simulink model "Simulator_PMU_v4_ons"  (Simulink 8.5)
settings: Solver=FixedStepDiscrete  StartTime=0.0  StopTime=5  FixedStep=1/(60*32)  RelTol=1e-3
undefined symbols (not defined in the file or in its folder): complex, j
libraries: dspxfrm3 x3

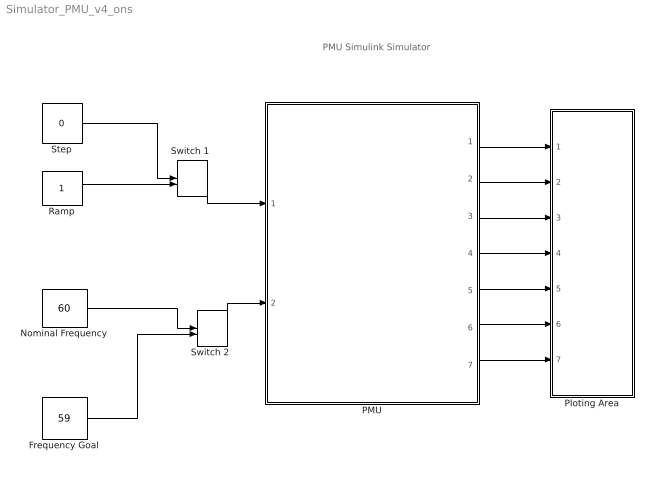
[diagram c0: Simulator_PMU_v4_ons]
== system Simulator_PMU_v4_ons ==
  note: PMU Simulink Simulator
  Frequency Goal : Constant  Value=59
  Nominal Frequency : Constant  Value=60
  PMU : Subsystem
  Ploting Area : Subsystem
  Ramp : Constant
  Step : Constant  Value=0
  "Switch 1 " : ManualSwitch
  "Switch 2 " : ManualSwitch  CurrentSetting=0
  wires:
  PMU/1(SP_MF) -> Ploting Area/1(SP_MF)
  PMU/2(SP_MnF) -> Ploting Area/2(SP_MnF)
  PMU/4(PS_Md) -> Ploting Area/4(PS_Md)
  PMU/6(PS_Ad) -> Ploting Area/6(PS_Ad)
  Step/1 -> "Switch 1 "/1
  Ramp/1 -> "Switch 1 "/2
  "Switch 2 "/1 -> PMU/2(Frequency Goal)
  PMU/3(PS_M) -> Ploting Area/3(PS_M)
  PMU/5(PS_A) -> Ploting Area/5(PS_A)
  PMU/7(Frequency  Deviation) -> Ploting Area/7(FD)
  Nominal Frequency/1 -> "Switch 2 "/1
  Frequency Goal/1 -> "Switch 2 "/2
  "Switch 1 "/1 -> PMU/1(Disturbance)

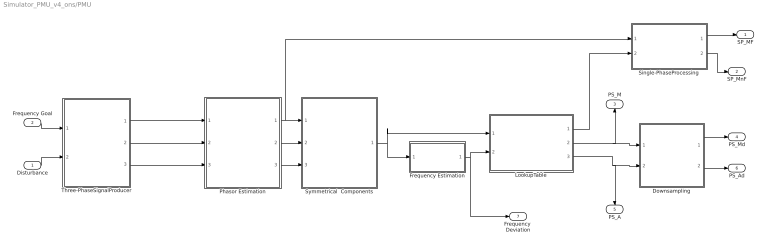
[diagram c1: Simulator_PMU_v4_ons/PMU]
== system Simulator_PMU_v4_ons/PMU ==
  Disturbance : Inport
  Frequency Goal : Inport  Port=2
  Downsampling : Subsystem
  Frequency Estimation : Subsystem
  LookupTable : Subsystem
  Phasor Estimation : Subsystem
  Single-PhaseProcessing : Subsystem
  Symmetrical  Components : Subsystem
  Three-PhaseSignalProducer : Subsystem
  SP_MF : Outport
  SP_MnF : Outport  Port=2
  PS_M : Outport  Port=3
  PS_Md : Outport  Port=4
  PS_A : Outport  Port=5
  PS_Ad : Outport  Port=6
  Frequency  Deviation : Outport  Port=7
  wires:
  Phasor Estimation/1(Phasor A) -> Single-PhaseProcessing/1(Phasor A), Symmetrical  Components/1(Phasor A)
  Symmetrical  Components/1(P_PS) -> Frequency Estimation/1(P_PS), LookupTable/1(P_ PS)
  LookupTable/2(PS_M) -> Downsampling/1(PS_M), PS_M/1
  LookupTable/3(PS_A) -> Downsampling/2(PS_A), PS_A/1
  Frequency Estimation/1(FD) -> LookupTable/2(FD), Frequency  Deviation/1
  LookupTable/1(CF) -> Single-PhaseProcessing/2(CF)
  Phasor Estimation/2(Phasor B) -> Symmetrical  Components/2(Phasor B)
  Phasor Estimation/3(Phasor C) -> Symmetrical  Components/3(Phasor C)
  Single-PhaseProcessing/1(SP_MF) -> SP_MF/1
  Single-PhaseProcessing/2(SP_MnF) -> SP_MnF/1
  Downsampling/1(" PS_Md") -> PS_Md/1
  Frequency Goal/1 -> Three-PhaseSignalProducer/1(Frequency)
  Downsampling/2(PS_Ad) -> PS_Ad/1
  Disturbance/1 -> Three-PhaseSignalProducer/2(Type)
  Three-PhaseSignalProducer/1(Phase A) -> Phasor Estimation/1(" Phase A")
  Three-PhaseSignalProducer/2(Phase B) -> Phasor Estimation/2(Phase B)
  Three-PhaseSignalProducer/3(Phase C) -> Phasor Estimation/3(Phase C)

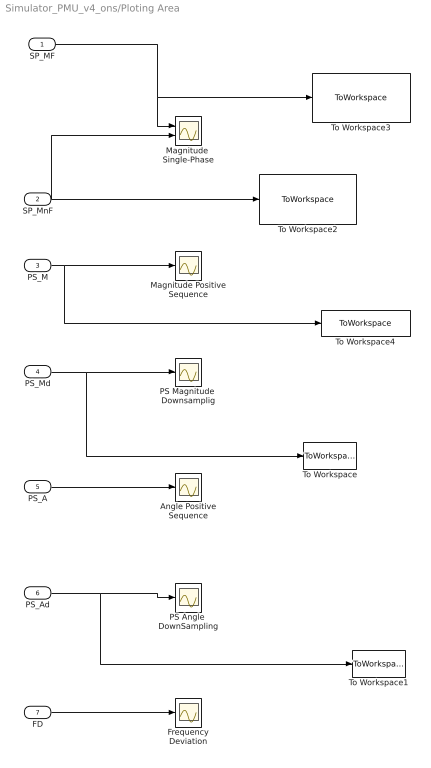
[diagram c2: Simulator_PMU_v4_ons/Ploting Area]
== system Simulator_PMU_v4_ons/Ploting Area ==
  SP_MF : Inport
  SP_MnF : Inport  Port=2
  PS_M : Inport  Port=3
  PS_Md : Inport  Port=4
  PS_A : Inport  Port=5
  PS_Ad : Inport  Port=6
  FD : Inport  Port=7
  Angle Positive Sequence : Scope
  Frequency Deviation : Scope
  Magnitude  Single-Phase : Scope  NumInputPorts=2
  Magnitude Positive Sequence : Scope
  PS Angle  DownSampling : Scope
  PS Magnitude  Downsamplig : Scope
  To Workspace : ToWorkspace  VariableName=simoutmagd  SaveFormat=Structure With Time  SampleTime=-1
  To Workspace1 : ToWorkspace  VariableName=simoutangd  SaveFormat=Structure With Time  SampleTime=-1
  To Workspace2 : ToWorkspace  VariableName=sp_mag_f  SaveFormat=Structure  SampleTime=-1
  To Workspace3 : ToWorkspace  VariableName=sp_mag  SaveFormat=Structure  SampleTime=-1
  To Workspace4 : ToWorkspace  VariableName=ps_magnitude  SaveFormat=Structure With Time  SampleTime=-1
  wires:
  SP_MF/1 -> Magnitude  Single-Phase/1, To Workspace3/1
  SP_MnF/1 -> Magnitude  Single-Phase/2, To Workspace2/1
  PS_M/1 -> Magnitude Positive Sequence/1, To Workspace4/1
  PS_Md/1 -> PS Magnitude  Downsamplig/1, To Workspace/1
  PS_A/1 -> Angle Positive Sequence/1
  PS_Ad/1 -> PS Angle  DownSampling/1, To Workspace1/1
  FD/1 -> Frequency Deviation/1

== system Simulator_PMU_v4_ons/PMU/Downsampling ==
  PS_M : Inport
  PS_A : Inport  Port=2
  Downsample A : DownSample  N=32  RateOptions=Allow multirate processing
  Downsample M : DownSample  N=32  RateOptions=Allow multirate processing
  Gain : Gain  Gain=180/pi
  " PS_Md" : Outport
  PS_Ad : Outport  Port=2
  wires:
  Downsample M/1 -> " PS_Md"/1
  PS_M/1 -> Downsample M/1
  PS_A/1 -> Downsample A/1
  Gain/1 -> PS_Ad/1
  Downsample A/1 -> Gain/1

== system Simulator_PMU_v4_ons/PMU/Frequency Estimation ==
  P_PS : Inport
  Complex to Magnitude-Angle : ComplexToMagnitudeAngle  Output=Angle
  Frequency Buffer : Buffer  N=32*2+1  V=32*2-1  TreatMby1Signals=One channel
  Frequency Datalog : ToWorkspace  VariableName=simoutf  SampleTime=-1
  Frequency  Estimation : MATLABFcn  MATLABFcn=freq_angle  Output1D=off
  FD : Outport
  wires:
  Frequency Buffer/1 -> Frequency  Estimation/1
  Frequency  Estimation/1 -> Frequency Datalog/1, FD/1
  Complex to Magnitude-Angle/1 -> Frequency Buffer/1
  P_PS/1 -> Complex to Magnitude-Angle/1

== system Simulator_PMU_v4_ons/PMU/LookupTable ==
  P_ PS : Inport
  FD : Inport  Port=2
  Complex to Magnitude-Angle : ComplexToMagnitudeAngle
  Divide : Product  Inputs=*/
  P_n Estimation : Subsystem
  Reshape : Reshape
  CF : Outport
  PS_M : Outport  Port=2
  PS_A : Outport  Port=3
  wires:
  Divide/1 -> Complex to Magnitude-Angle/1
  FD/1 -> Reshape/1
  Complex to Magnitude-Angle/1 -> PS_M/1
  Complex to Magnitude-Angle/2 -> PS_A/1
  P_ PS/1 -> Divide/1
  P_n Estimation/1(P_n) -> Divide/2, CF/1
  Reshape/1 -> P_n Estimation/1(Frequency Deviation)

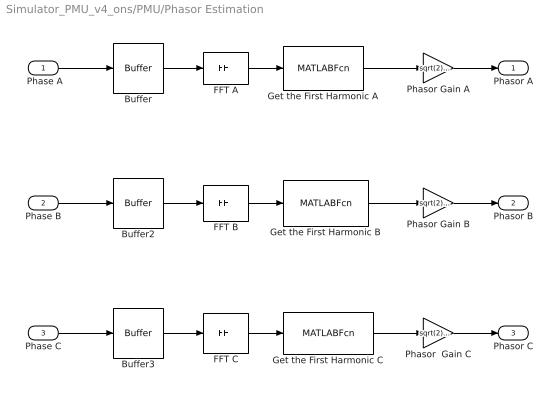
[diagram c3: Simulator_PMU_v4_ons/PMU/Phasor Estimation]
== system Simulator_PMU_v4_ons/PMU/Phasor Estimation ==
  " Phase A" : Inport
  Phase B : Inport  Port=2
  Phase C : Inport  Port=3
  Buffer : Buffer  N=32  V=31  TreatMby1Signals=One channel
  Buffer2 : Buffer  N=32  V=31  TreatMby1Signals=One channel
  Buffer3 : Buffer  N=32  V=31  TreatMby1Signals=One channel
  FFT A : dspxfrm3/FFT  CompMethod=Table lookup  TableOpt=HYBRID  TableOptActive=Speed  BitRevOrder=off  InheritFFTLength=on  FFTLength=31  WrapInput=on  RowConvenienceOn=on  FFTImplementation=Auto  SkipNorm=off  firstCoeffDataTypeStr=Inherit: Same word length as input  firstCoeffLastDataTypeStr=Inherit: Same word length as input  outputMin=[]  outputMax=[]  roundingMode=Round  overflowMode=off
  FFT B : dspxfrm3/FFT  CompMethod=Table lookup  TableOpt=HYBRID  TableOptActive=Speed  BitRevOrder=off  InheritFFTLength=on  FFTLength=32  WrapInput=on  RowConvenienceOn=on  FFTImplementation=Auto  SkipNorm=off  firstCoeffDataTypeStr=Inherit: Same word length as input  firstCoeffLastDataTypeStr=Inherit: Same word length as input  outputMin=[]  outputMax=[]  roundingMode=Round  overflowMode=off
  FFT C : dspxfrm3/FFT  CompMethod=Table lookup  TableOpt=HYBRID  TableOptActive=Speed  BitRevOrder=off  InheritFFTLength=on  FFTLength=32  WrapInput=on  RowConvenienceOn=on  FFTImplementation=Auto  SkipNorm=off  firstCoeffDataTypeStr=Inherit: Same word length as input  firstCoeffLastDataTypeStr=Inherit: Same word length as input  outputMin=[]  outputMax=[]  roundingMode=Round  overflowMode=off
  Get the First Harmonic A : MATLABFcn  MATLABFcn=u(2,1,1)  OutputSignalType=complex
  Get the First Harmonic B : MATLABFcn  MATLABFcn=u(2,1,1)  OutputSignalType=complex
  Get the First Harmonic C : MATLABFcn  MATLABFcn=u(2,1,1)  OutputSignalType=complex
  Phasor Gain A : Gain  Gain=sqrt(2)/32
  Phasor Gain B : Gain  Gain=sqrt(2)/32
  Phasor  Gain C : Gain  Gain=sqrt(2)/32
  Phasor A : Outport
  Phasor B : Outport  Port=2
  Phasor C : Outport  Port=3
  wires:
  FFT A/1 -> Get the First Harmonic A/1
  Buffer/1 -> FFT A/1
  Get the First Harmonic A/1 -> Phasor Gain A/1
  FFT B/1 -> Get the First Harmonic B/1
  Buffer2/1 -> FFT B/1
  Get the First Harmonic B/1 -> Phasor Gain B/1
  FFT C/1 -> Get the First Harmonic C/1
  Buffer3/1 -> FFT C/1
  Get the First Harmonic C/1 -> Phasor  Gain C/1
  " Phase A"/1 -> Buffer/1
  Phasor Gain A/1 -> Phasor A/1
  Phase B/1 -> Buffer2/1
  Phasor Gain B/1 -> Phasor B/1
  Phase C/1 -> Buffer3/1
  Phasor  Gain C/1 -> Phasor C/1

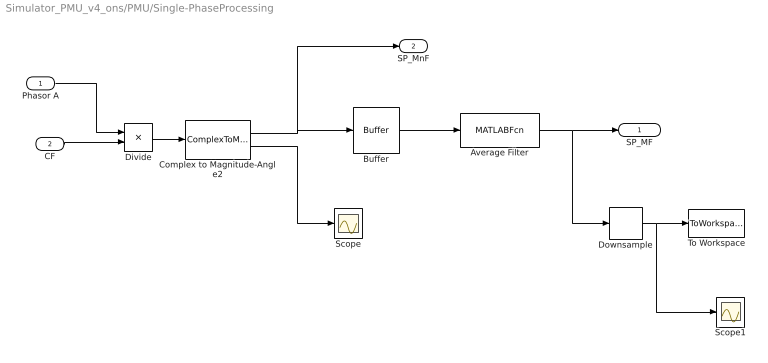
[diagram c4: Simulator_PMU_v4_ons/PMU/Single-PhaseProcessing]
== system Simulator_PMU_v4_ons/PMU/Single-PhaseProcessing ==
  Phasor A : Inport
  CF : Inport  Port=2
  Average Filter : MATLABFcn  MATLABFcn=( u(1)+u(6)+u(12) )/3  Output1D=off
  Buffer : Buffer  N=32  V=31  TreatMby1Signals=One channel
  Complex to Magnitude-Angle2 : ComplexToMagnitudeAngle
  Divide : Product  Inputs=*/
  Downsample : DownSample  N=32  RateOptions=Allow multirate processing
  Scope : Scope
  Scope1 : Scope
  To Workspace : ToWorkspace  VariableName=single  SaveFormat=Structure  SampleTime=-1
  SP_MF : Outport
  SP_MnF : Outport  Port=2
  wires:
  Phasor A/1 -> Divide/1
  CF/1 -> Divide/2
  Complex to Magnitude-Angle2/2 -> Scope/1
  Complex to Magnitude-Angle2/1 -> Buffer/1, SP_MnF/1
  Buffer/1 -> Average Filter/1
  Divide/1 -> Complex to Magnitude-Angle2/1
  Average Filter/1 -> SP_MF/1, Downsample/1
  Downsample/1 -> To Workspace/1, Scope1/1

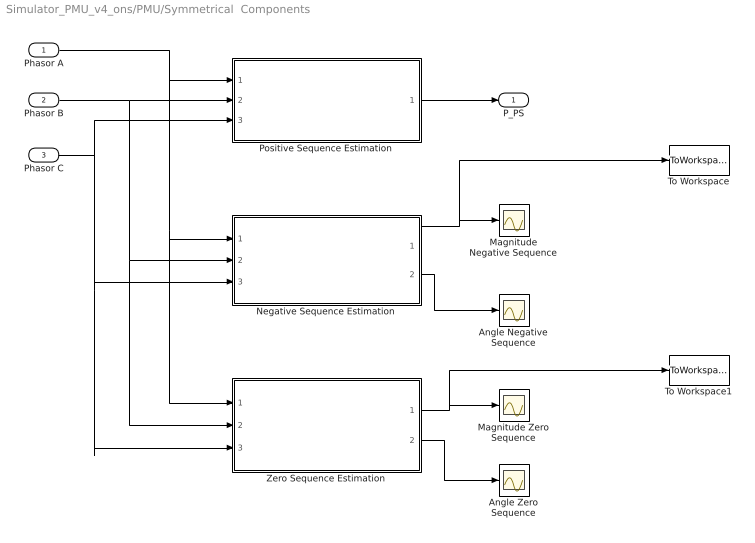
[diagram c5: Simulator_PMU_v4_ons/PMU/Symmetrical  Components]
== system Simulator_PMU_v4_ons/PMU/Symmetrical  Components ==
  Phasor A : Inport
  Phasor B : Inport  Port=2
  Phasor C : Inport  Port=3
  Angle Negative Sequence : Scope
  Angle Zero Sequence : Scope
  Magnitude Negative Sequence : Scope
  Magnitude Zero Sequence : Scope
  Negative Sequence Estimation : Subsystem
  Positive Sequence Estimation : Subsystem
  To Workspace : ToWorkspace  VariableName=negative  SaveFormat=Structure  SampleTime=-1
  To Workspace1 : ToWorkspace  VariableName=zero  SaveFormat=Structure  SampleTime=-1
  Zero Sequence Estimation : Subsystem
  P_PS : Outport
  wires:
  Phasor C/1 -> Zero Sequence Estimation/3(Phasor C), Negative Sequence Estimation/3(Phasor C), Positive Sequence Estimation/3(Phasor C)
  Phasor B/1 -> Zero Sequence Estimation/2(Phasor B), Negative Sequence Estimation/2(Phasor B), Positive Sequence Estimation/2(Phasor B)
  Negative Sequence Estimation/2(Angle) -> Angle Negative Sequence/1
  Negative Sequence Estimation/1(Magnitude) -> Magnitude Negative Sequence/1, To Workspace/1
  Zero Sequence Estimation/2(Angle) -> Angle Zero Sequence/1
  Zero Sequence Estimation/1(Magnitude) -> Magnitude Zero Sequence/1, To Workspace1/1
  Phasor A/1 -> Positive Sequence Estimation/1(Phasor A), Negative Sequence Estimation/1(Phasor A), Zero Sequence Estimation/1(Phasor A)
  Positive Sequence Estimation/1(Positive Sequence) -> P_PS/1

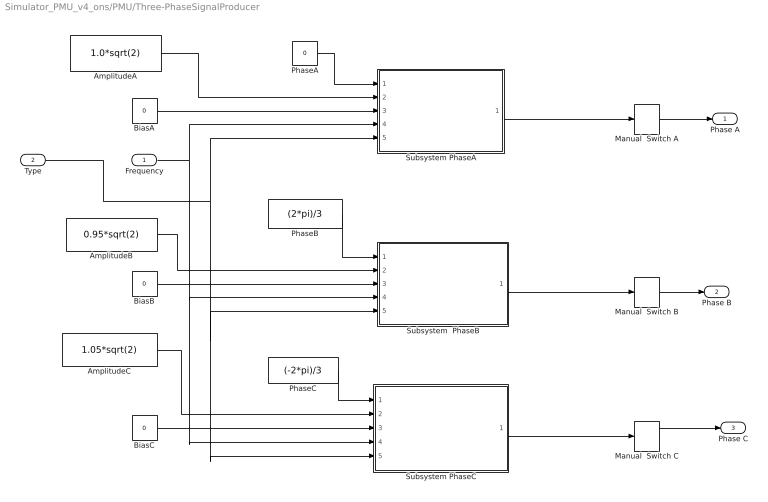
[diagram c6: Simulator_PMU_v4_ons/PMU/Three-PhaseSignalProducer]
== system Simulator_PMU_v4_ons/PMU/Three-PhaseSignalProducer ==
  Frequency : Inport
  Type : Inport  Port=2
  AmplitudeA : Constant  Value=1.0*sqrt(2)
  AmplitudeB : Constant  Value=0.95*sqrt(2)
  AmplitudeC : Constant  Value=1.05*sqrt(2)
  BiasA : Constant  Value=0
  BiasB : Constant  Value=0
  BiasC : Constant  Value=0
  Manual  Switch A : ManualSwitch
  Manual  Switch B : ManualSwitch
  Manual  Switch C : ManualSwitch
  PhaseA : Constant  Value=0
  PhaseB : Constant  Value=(2*pi)/3
  PhaseC : Constant  Value=(-2*pi)/3
  Subsystem PhaseA : Subsystem
  Subsystem PhaseC : Subsystem
  Subsystem  PhaseB : Subsystem
  Phase A : Outport
  Phase B : Outport  Port=2
  Phase C : Outport  Port=3
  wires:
  AmplitudeB/1 -> Subsystem  PhaseB/2(Amplitude)
  BiasB/1 -> Subsystem  PhaseB/3(Bias)
  PhaseB/1 -> Subsystem  PhaseB/1(Phase)
  AmplitudeC/1 -> Subsystem PhaseC/2(Amplitude)
  BiasC/1 -> Subsystem PhaseC/3(Bias)
  PhaseC/1 -> Subsystem PhaseC/1(Phase)
  BiasA/1 -> Subsystem PhaseA/3(Bias)
  PhaseA/1 -> Subsystem PhaseA/1(Phase)
  AmplitudeA/1 -> Subsystem PhaseA/2(Amplitude)
  Frequency/1 -> Subsystem PhaseA/4(Frequency), Subsystem  PhaseB/4(Frequency), Subsystem PhaseC/4(Frequency)
  Type/1 -> Subsystem PhaseA/5(Ramp/Step), Subsystem  PhaseB/5(Ramp/Step), Subsystem PhaseC/5(Ramp/Step)
  Subsystem PhaseC/1(Signal) -> Manual  Switch C/1
  Manual  Switch C/1 -> Phase C/1
  Manual  Switch B/1 -> Phase B/1
  Subsystem  PhaseB/1(Signal) -> Manual  Switch B/1
  Manual  Switch A/1 -> Phase A/1
  Subsystem PhaseA/1("Signal ") -> Manual  Switch A/1

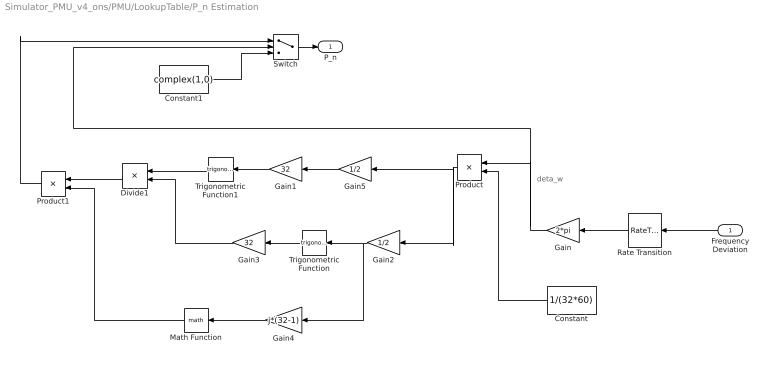
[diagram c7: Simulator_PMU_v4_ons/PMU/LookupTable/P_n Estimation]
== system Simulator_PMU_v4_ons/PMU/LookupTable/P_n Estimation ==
  note: deta_w
  Frequency Deviation : Inport
  Constant : Constant  Value=1/(32*60)
  Constant1 : Constant  Value=complex(1,0)  VectorParams1D=off
  Divide1 : Product  Inputs=*/
  Gain : Gain  Gain=2*pi  SampleTime=1/(32*60)
  Gain1 : Gain  Gain=32
  Gain2 : Gain  Gain=1/2
  Gain3 : Gain  Gain=32
  Gain4 : Gain  Gain=j*(32-1)
  Gain5 : Gain  Gain=1/2
  Math Function : Math
  Product : Product
  Product1 : Product
  Rate Transition : RateTransition  OutPortSampleTime=1/(32*60)
  Switch : Switch  Criteria=u2 ~= 0
  Trigonometric Function : Trigonometry
  Trigonometric Function1 : Trigonometry
  P_n : Outport
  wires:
  Gain/1 -> Product/1, Switch/2
  Constant/1 -> Product/2
  Product/1 -> Gain2/1, Gain5/1
  Gain2/1 -> Trigonometric Function/1, Gain4/1
  Trigonometric Function/1 -> Gain3/1
  Gain1/1 -> Trigonometric Function1/1
  Gain3/1 -> Divide1/2
  Trigonometric Function1/1 -> Divide1/1
  Gain4/1 -> Math Function/1
  Product1/1 -> Switch/1
  Constant1/1 -> Switch/3
  Gain5/1 -> Gain1/1
  Rate Transition/1 -> Gain/1
  Divide1/1 -> Product1/1
  Math Function/1 -> Product1/2
  Switch/1 -> P_n/1
  Frequency Deviation/1 -> Rate Transition/1

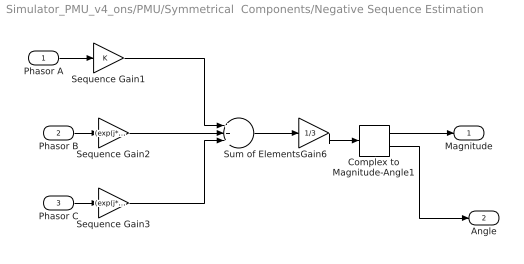
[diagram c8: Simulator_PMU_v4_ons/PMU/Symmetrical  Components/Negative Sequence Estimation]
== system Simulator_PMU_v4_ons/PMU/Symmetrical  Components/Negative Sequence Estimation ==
  Phasor A : Inport
  Phasor B : Inport  Port=2
  Phasor C : Inport  Port=3
  Complex to Magnitude-Angle1 : ComplexToMagnitudeAngle
  Gain6 : Gain  Gain=1/3  SampleTime=1/(32*60)
  Sequence Gain1 : Gain
  Sequence Gain2 : Gain  Gain=(exp(j*2*pi/3))
  Sequence Gain3 : Gain  Gain=(exp(j*2*pi/3))^2
  Sum of Elements : Sum  Inputs=+++
  Magnitude : Outport
  Angle : Outport  Port=2
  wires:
  Sequence Gain1/1 -> Sum of Elements/1
  Sequence Gain2/1 -> Sum of Elements/2
  Sequence Gain3/1 -> Sum of Elements/3
  Sum of Elements/1 -> Gain6/1
  Phasor A/1 -> Sequence Gain1/1
  Gain6/1 -> Complex to Magnitude-Angle1/1
  Phasor B/1 -> Sequence Gain2/1
  Phasor C/1 -> Sequence Gain3/1
  Complex to Magnitude-Angle1/1 -> Magnitude/1
  Complex to Magnitude-Angle1/2 -> Angle/1

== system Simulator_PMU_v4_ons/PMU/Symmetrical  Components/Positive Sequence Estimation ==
  Phasor A : Inport
  Phasor B : Inport  Port=2
  Phasor C : Inport  Port=3
  Gain6 : Gain  Gain=1/3  SampleTime=1/(32*60)
  Sequence Gain1 : Gain
  Sequence Gain2 : Gain  Gain=(exp(j*2*pi/3))^2
  Sequence Gain3 : Gain  Gain=exp(j*2*pi/3)
  Sum of Elements : Sum  Inputs=+++
  Positive Sequence : Outport
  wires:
  Sequence Gain1/1 -> Sum of Elements/1
  Sequence Gain2/1 -> Sum of Elements/2
  Sequence Gain3/1 -> Sum of Elements/3
  Sum of Elements/1 -> Gain6/1
  Phasor A/1 -> Sequence Gain1/1
  Gain6/1 -> Positive Sequence/1
  Phasor B/1 -> Sequence Gain2/1
  Phasor C/1 -> Sequence Gain3/1

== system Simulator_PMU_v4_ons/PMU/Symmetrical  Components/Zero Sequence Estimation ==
  Phasor A : Inport
  Phasor B : Inport  Port=2
  Phasor C : Inport  Port=3
  Complex to Magnitude-Angle1 : ComplexToMagnitudeAngle
  Gain6 : Gain  Gain=1/3  SampleTime=1/(32*60)
  Sequence Gain1 : Gain
  Sequence Gain2 : Gain
  Sequence Gain3 : Gain
  Sum of Elements : Sum  Inputs=+++
  Magnitude : Outport
  Angle : Outport  Port=2
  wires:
  Sequence Gain1/1 -> Sum of Elements/1
  Sequence Gain2/1 -> Sum of Elements/2
  Sequence Gain3/1 -> Sum of Elements/3
  Sum of Elements/1 -> Gain6/1
  Phasor A/1 -> Sequence Gain1/1
  Gain6/1 -> Complex to Magnitude-Angle1/1
  Phasor B/1 -> Sequence Gain2/1
  Phasor C/1 -> Sequence Gain3/1
  Complex to Magnitude-Angle1/1 -> Magnitude/1
  Complex to Magnitude-Angle1/2 -> Angle/1

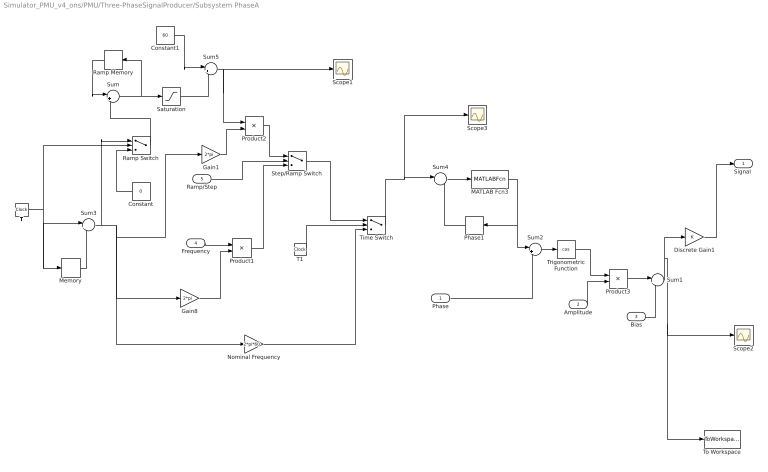
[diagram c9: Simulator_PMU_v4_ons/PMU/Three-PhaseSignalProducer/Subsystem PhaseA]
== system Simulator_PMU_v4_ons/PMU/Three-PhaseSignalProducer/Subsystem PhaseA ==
  Phase : Inport
  Amplitude : Inport  Port=2
  Bias : Inport  Port=3
  Frequency : Inport  Port=4
  Ramp/Step : Inport  Port=5
  Constant : Constant  Value=0
  Constant1 : Constant  Value=60
  Discrete Gain1 : Gain  SampleTime=1/(32*60)
  Gain1 : Gain  Gain=2*pi
  Gain8 : Gain  Gain=2*pi
  MATLAB Fcn3 : MATLABFcn  MATLABFcn=rem(u,2*pi)
  Memory : Memory
  Nominal Frequency : Gain  Gain=2*pi*60
  Phase1 : Memory  X0=-(2*pi)/32  LinearizeMemory=on
  Product1 : Product
  Product2 : Product
  Product3 : Product
  Ramp Memory : Memory
  Ramp Switch : Switch  Threshold=2
  Saturation : Saturate  UpperLimit=1  LowerLimit=-1
  Scope1 : Scope
  Scope2 : Scope
  Scope3 : Scope
  Step/Ramp Switch : Switch  Criteria=u2 ~= 0  Threshold=2
  Sum : Sum  Inputs=|+-
  Sum{1..2,4..5} (4 alike) : Sum  Inputs=|++
  Sum3 : Sum  Inputs=|+-
  T : Clock
  T1 : Clock
  Time Switch : Switch  Threshold=2
  To Workspace : ToWorkspace  VariableName=simout1  SaveFormat=Structure  SampleTime=-1
  Trigonometric Function : Trigonometry  Operator=cos
  "Signal " : Outport
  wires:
  Trigonometric Function/1 -> Product3/1
  Product3/1 -> Sum1/1
  T/1 -> Memory/1, Sum3/1, Ramp Switch/2
  Sum3/1 -> Ramp Switch/1, Nominal Frequency/1, Gain8/1, Gain1/1
  Phase1/1 -> Sum4/2
  Sum4/1 -> MATLAB Fcn3/1
  MATLAB Fcn3/1 -> Phase1/1, Sum2/1
  Nominal Frequency/1 -> Time Switch/3
  Time Switch/1 -> Sum4/1, Scope3/1
  Sum/1 -> Ramp Memory/1, Saturation/1
  Ramp Memory/1 -> Sum/1
  Ramp Switch/1 -> Sum/2
  Constant/1 -> Ramp Switch/3
  Product2/1 -> Step/Ramp Switch/1
  Step/Ramp Switch/1 -> Time Switch/1
  T1/1 -> Time Switch/2
  Memory/1 -> Sum3/2
  Sum2/1 -> Trigonometric Function/1
  Phase/1 -> Sum2/2
  Amplitude/1 -> Product3/2
  Bias/1 -> Sum1/2
  Discrete Gain1/1 -> "Signal "/1
  Sum1/1 -> Discrete Gain1/1, Scope2/1, To Workspace/1
  Gain8/1 -> Product1/2
  Product1/1 -> Step/Ramp Switch/3
  Frequency/1 -> Product1/1
  Ramp/Step/1 -> Step/Ramp Switch/2
  Sum5/1 -> Product2/1, Scope1/1
  Saturation/1 -> Sum5/2
  Constant1/1 -> Sum5/1
  Gain1/1 -> Product2/2

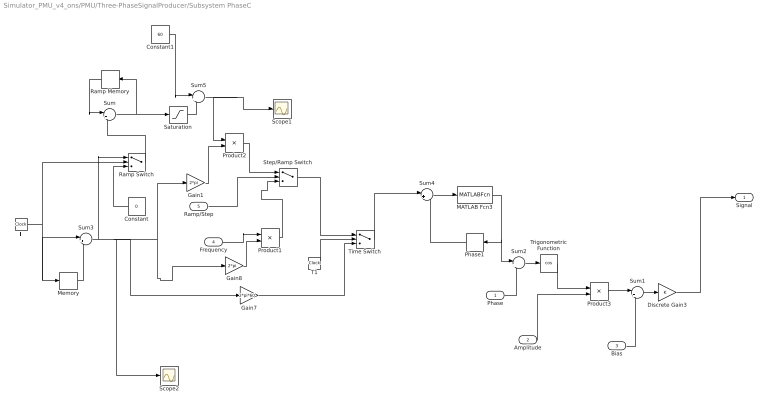
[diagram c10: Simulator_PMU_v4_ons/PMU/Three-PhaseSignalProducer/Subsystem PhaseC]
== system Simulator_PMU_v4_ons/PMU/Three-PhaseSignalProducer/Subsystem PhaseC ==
  Phase : Inport
  Amplitude : Inport  Port=2
  Bias : Inport  Port=3
  Frequency : Inport  Port=4
  Ramp/Step : Inport  Port=5
  Constant : Constant  Value=0
  Constant1 : Constant  Value=60
  Discrete Gain3 : Gain  SampleTime=1/(32*60)
  Gain1 : Gain  Gain=2*pi
  Gain7 : Gain  Gain=2*pi*60
  Gain8 : Gain  Gain=2*pi
  MATLAB Fcn3 : MATLABFcn  MATLABFcn=rem(u,2*pi)
  Memory : Memory
  Phase1 : Memory  X0=-(2*pi)/32
  Product1 : Product
  Product2 : Product
  Product3 : Product
  Ramp Memory : Memory
  Ramp Switch : Switch  Threshold=2
  Saturation : Saturate  UpperLimit=1  LowerLimit=-1
  Scope1 : Scope
  Scope2 : Scope
  Step/Ramp Switch : Switch  Criteria=u2 ~= 0  Threshold=2
  Sum : Sum  Inputs=|+-
  Sum{1..2,4..5} (4 alike) : Sum  Inputs=|++
  Sum3 : Sum  Inputs=|+-
  T : Clock
  T1 : Clock
  Time Switch : Switch  Threshold=2
  Trigonometric Function : Trigonometry  Operator=cos
  Signal : Outport
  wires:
  Trigonometric Function/1 -> Product3/1
  Product3/1 -> Sum1/1
  T/1 -> Memory/1, Sum3/1, Ramp Switch/2
  Sum3/1 -> Ramp Switch/1, Gain7/1, Gain8/1, Gain1/1, Scope2/1
  Phase1/1 -> Sum4/2
  Sum4/1 -> MATLAB Fcn3/1
  MATLAB Fcn3/1 -> Phase1/1, Sum2/1
  Gain7/1 -> Time Switch/3
  Time Switch/1 -> Sum4/1
  Sum/1 -> Ramp Memory/1, Saturation/1
  Ramp Memory/1 -> Sum/1
  Ramp Switch/1 -> Sum/2
  Constant/1 -> Ramp Switch/3
  Product2/1 -> Step/Ramp Switch/1
  Step/Ramp Switch/1 -> Time Switch/1
  T1/1 -> Time Switch/2
  Memory/1 -> Sum3/2
  Sum2/1 -> Trigonometric Function/1
  Phase/1 -> Sum2/2
  Amplitude/1 -> Product3/2
  Bias/1 -> Sum1/2
  Sum1/1 -> Discrete Gain3/1
  Discrete Gain3/1 -> Signal/1
  Product1/1 -> Step/Ramp Switch/3
  Frequency/1 -> Product1/1
  Gain8/1 -> Product1/2
  Ramp/Step/1 -> Step/Ramp Switch/2
  Saturation/1 -> Sum5/2
  Sum5/1 -> Scope1/1, Product2/1
  Constant1/1 -> Sum5/1
  Gain1/1 -> Product2/2

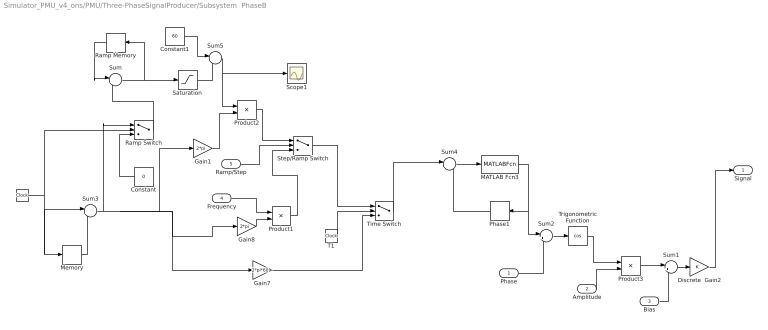
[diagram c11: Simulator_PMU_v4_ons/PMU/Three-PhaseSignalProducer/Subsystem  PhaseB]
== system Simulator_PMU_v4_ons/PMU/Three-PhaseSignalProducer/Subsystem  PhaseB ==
  Phase : Inport
  Amplitude : Inport  Port=2
  Bias : Inport  Port=3
  Frequency : Inport  Port=4
  Ramp/Step : Inport  Port=5
  Constant : Constant  Value=0
  Constant1 : Constant  Value=60
  Discrete  Gain2 : Gain  SampleTime=1/(32*60)
  Gain1 : Gain  Gain=2*pi
  Gain7 : Gain  Gain=2*pi*60
  Gain8 : Gain  Gain=2*pi
  MATLAB Fcn3 : MATLABFcn  MATLABFcn=rem(u,2*pi)
  Memory : Memory
  Phase1 : Memory  X0=-(2*pi)/32
  Product1 : Product
  Product2 : Product
  Product3 : Product
  Ramp Memory : Memory
  Ramp Switch : Switch  Threshold=2
  Saturation : Saturate  UpperLimit=1  LowerLimit=-1
  Scope1 : Scope
  Step/Ramp Switch : Switch  Criteria=u2 ~= 0  Threshold=2
  Sum : Sum  Inputs=|+-
  Sum{1..2,4..5} (4 alike) : Sum  Inputs=|++
  Sum3 : Sum  Inputs=|+-
  T : Clock
  T1 : Clock
  Time Switch : Switch  Threshold=2
  Trigonometric Function : Trigonometry  Operator=cos
  Signal : Outport
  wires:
  Trigonometric Function/1 -> Product3/1
  Product3/1 -> Sum1/1
  T/1 -> Memory/1, Sum3/1, Ramp Switch/2
  Sum3/1 -> Ramp Switch/1, Gain7/1, Gain8/1, Gain1/1
  Phase1/1 -> Sum4/2
  Sum4/1 -> MATLAB Fcn3/1
  MATLAB Fcn3/1 -> Phase1/1, Sum2/1
  Gain7/1 -> Time Switch/3
  Time Switch/1 -> Sum4/1
  Sum/1 -> Ramp Memory/1, Saturation/1
  Ramp Memory/1 -> Sum/1
  Ramp Switch/1 -> Sum/2
  Constant/1 -> Ramp Switch/3
  Product2/1 -> Step/Ramp Switch/1
  Step/Ramp Switch/1 -> Time Switch/1
  T1/1 -> Time Switch/2
  Memory/1 -> Sum3/2
  Sum2/1 -> Trigonometric Function/1
  Phase/1 -> Sum2/2
  Amplitude/1 -> Product3/2
  Bias/1 -> Sum1/2
  Discrete  Gain2/1 -> Signal/1
  Sum1/1 -> Discrete  Gain2/1
  Product1/1 -> Step/Ramp Switch/3
  Frequency/1 -> Product1/1
  Gain8/1 -> Product1/2
  Ramp/Step/1 -> Step/Ramp Switch/2
  Saturation/1 -> Sum5/2
  Sum5/1 -> Product2/1, Scope1/1
  Constant1/1 -> Sum5/1
  Gain1/1 -> Product2/2
